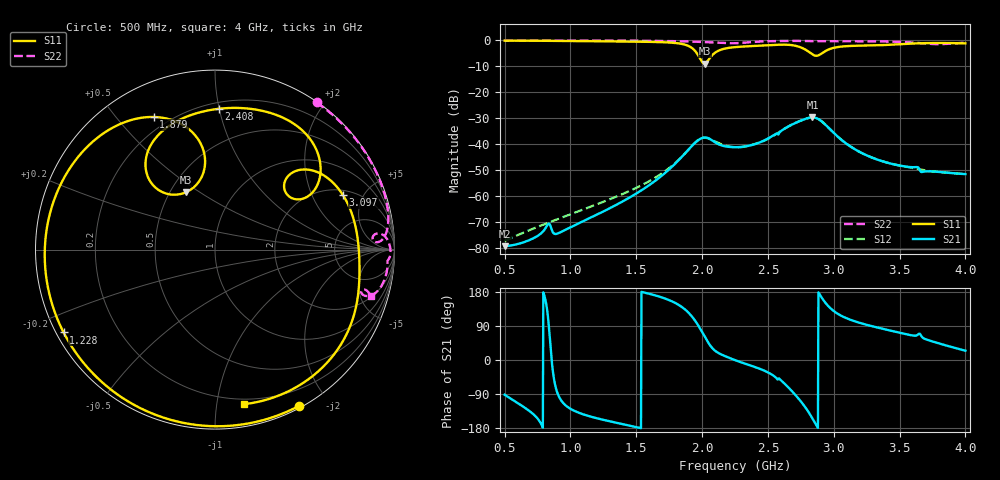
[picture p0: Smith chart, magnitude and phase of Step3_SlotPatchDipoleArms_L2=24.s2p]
! TOUCHSTONE file generated by CST MICROWAVE STUDIO
! Date and time: Mon May 18 03:17:24 2020
! Project name: DualBand_DualMode_Antenna_FD_SteppedDesign.cst
! Parameters = {FPL=20; FPW=20; L=50; ST=10; SW=30; W=52; WF=7; ext=10; gap=1; inset=13}
! Header version: 2015
! Port assignment regex: !\s*Touchstone port\s*([0-9]+)\s*=\s*CST MWS port\s*([0-9]+)\s*\(\"(.*)\"\)(\s*mode\s*([0-9]+))?.*
! Touchstone port assignment:
! Touchstone port 1 = CST MWS port 1 ("")
! Touchstone port 2 = CST MWS port 2 ("")
# GHz S MA R 50
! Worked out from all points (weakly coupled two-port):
!   1006 points, 500 MHz to 4 GHz, reference 50 ohm
!   highest |S21| = -29.63 dB at 2.838 GHz (marker M1); lowest = -79.2 dB at 500 MHz (marker M2)
!   lowest |S11| = -8.9 dB at 2.019 GHz (marker M3), VSWR 2.12, Z = 30 + j22 ohm
!   |S11| at or under -10 dB: nowhere
!   |S22| runs from -1.4 to 0.0 dB; largest |S21 - S12| = 0.0015
!   S11 on the Smith chart (normalised r, x): 500 MHz: 0.02, -1.68; 1.228 GHz: 0.02, -0.26; 1.879 GHz: 0.14, +0.63; 2.408 GHz: 0.24, +1.00; 3.097 GHz: 2.29, +3.48; 4 GHz: 0.16, -1.20
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0.5  0.9886 -61.6  0.0001102 -91.7  0.000139 -94.0  0.9963 55.4
0.787  0.9823 -96.9  0.0002053 -175.4  0.0002818 -122.3  0.9971 34.7
0.8325  0.9806 -102.6  0.0002974 102.7  0.0003123 -126.1  0.9971 32.5
0.899  0.9779 -110.8  0.0001917 -85.1  0.0003623 -131.6  0.997 29.6
1.0845  0.9692 -133.6  0.0003228 -141.9  0.0005444 -147.1  0.996 22.9
1.228  0.9616 -151.3  0.0004817 -156.1  0.0007482 -159.6  0.9943 18.7
1.4555  0.9484 -179.7  0.0009705 -173.6  0.001293 -179.6  0.9882 13.2
1.669  0.9282 151.7  0.002225 167.9  0.002507 161.0  0.9765 8.9
1.879  0.8139 114.8  0.007101 130.8  0.007059 129.1  0.9551 5.2
1.963  0.5526 96.6  0.01166 95.4  0.01176 95.8  0.9408 3.9
2.019  0.3581 116.8  0.01356 62.5  0.01344 63.0  0.9282 3.1
2.1065  0.598 130.3  0.01064 22.4  0.01113 25.3  0.9033 2.6
2.25  0.7416 108.3  0.008831 -0.3  0.008831 -0.3  0.8823 4.7
2.4075  0.7851 88.3  0.01021 -19.3  0.0103 -18.6  0.9402 5.0
2.705  0.792 44.4  0.02557 -90.8  0.02564 -90.6  0.9778 -1.0
2.8345  0.5456 30.9  0.03297 -152.0  0.03296 -152.0  0.9674 -3.3
2.838  0.5384 31.3  0.03298 -154.1  0.03297 -154.0  0.967 -3.3
2.9605  0.6678 42.0  0.02084 141.5  0.02086 141.5  0.9642 -4.6
3.097  0.7749 23.1  0.01028 110.2  0.01028 110.2  0.9654 -6.6
3.419  0.822 -12.0  0.004359 78.5  0.004366 78.4  0.9482 -12.5
3.671  0.8826 -40.4  0.002948 60.6  0.003232 58.7  0.8805 -17.1
4  0.8767 -79.2  0.002681 24.6  0.002681 24.6  0.9042 -16.6
